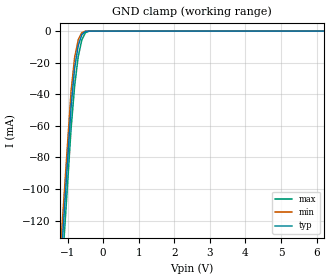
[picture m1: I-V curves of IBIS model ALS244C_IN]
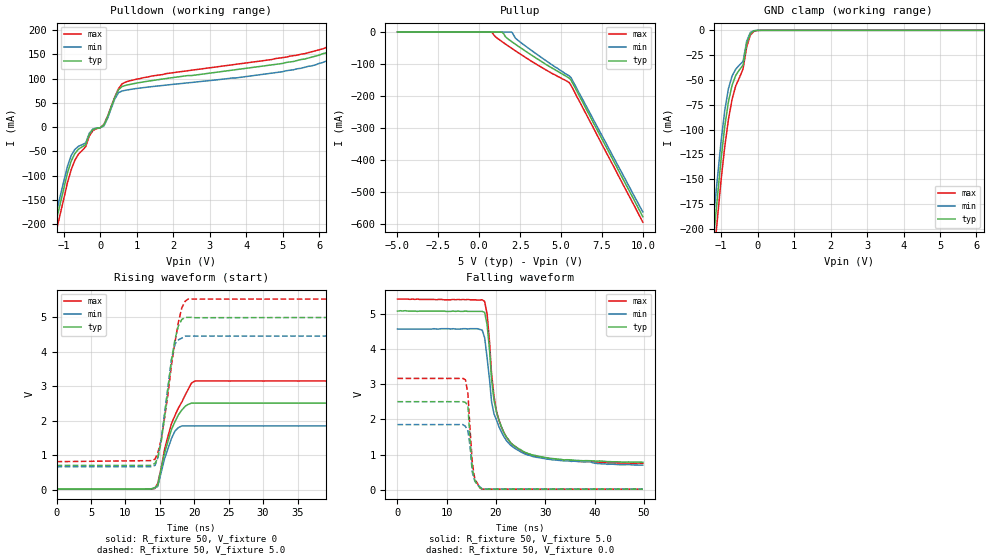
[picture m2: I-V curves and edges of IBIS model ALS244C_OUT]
| TEXAS INSTRUMENTS INCORPORATED
| Standard Linear and Logic Group
| IBIS Model of SN74ALS244C
| OCTAL BUFFERS AND LINE DRIVERS WITH 3-STATE OUTPUTS
| SOIC 20-pin (DW), SOP 20-pin (NS), SSOP 20-pin (DB), PDIP 20-pin (N) Package
[IBIS Ver]   3.2
[Comment Char]  |_char
[File Name]   sn74als244c.ibs
[File Rev]   3.1
[Date]   Sept. 23, 2004
[Source]   Data created from Labo data at TI-SLL.
[Notes]   The following is an IBIS list for the ALS244C.
   - FILE REV HISTORY
   - 3.1 Re-Release IBIS file on 09/23/04
   - Power clamp data deleted as there is no power-clamp diode
|   Please contact sllibis@ti.com with questions and
|   comments concerning SLL IBIS models.
[Disclaimer] Property of Texas Instruments Incorporated.  Unauthorized
   reproduction and/or distribution is strictly prohibited.
   This product is protected under copyright law.
   Created 2000, (C) Copyright 2000, Texas Instruments Inc.,
   All Rights Reserved.
   UNLESS THERE IS A SIGNED, WRITTEN AGREEMENT TO THE
   CONTRARY, TEXAS INSTRUMENTS () IS PROVIDING THE IBIS
   MODELS  AND WITHOUT ANY WARRANTY, EXPRESSED OR
   IMPLIED.  TI assumes no liability for:
   1) the accuracy of the IBIS models provided to your
   company;
   2) the proper functioning of these IBIS Models in your
   design or for any resulting applications; or
   3) infringement of patents, copyrights or intellectual
   property rights resulting from your use of these IBIS
   models.
   TI provides IBIS Models as a service to our customers.
   You and your company shall not distribute, sell or give
   these models to anyone else without prior written
   permission from TI.
   TI reserves the right to make changes to our products or
   to discontinue any semiconductor product or service
   without notice, and advises our customers to obtain the
   latest version of relevant information to verify, before
   placing orders, that the information being relied on is
   current.
   Please be aware that your receipt and use of the IBIS
   information provided shall serve as acceptance of these
   terms and conditions.  If you do not accept these terms,
   you should return or destroy the IBIS models and any
   other accompanying information immediately.
|   Component ALS244C_DW
[Component]   ALS244C_DW
[Manufacturer]  Texas Instruments, Inc.
[Package]
|   typ   min   max
R_pkg   0.038   0.033   0.045
L_pkg   5.012nH   4.110nH   6.349nH
C_pkg   0.717pF   0.530pF   0.868pF
[Pin]   signal_name   model_name   R_pin   L_pin   C_pin
1   1OE_NOT   ALS244C_IN   0.042   6.336nH   0.865pF
2   1A1   ALS244C_IN   0.043   5.542nH   0.867pF
3   2Y4   ALS244C_OUT   0.034   4.714nH   0.732pF
4   1A2   ALS244C_IN   0.034   4.377nH   0.591pF
5   2Y3   ALS244C_OUT   0.036   4.130nH   0.533pF
6   1A3   ALS244C_IN   0.035   4.111nH   0.530pF
7   2Y2   ALS244C_OUT   0.034   4.284nH   0.583pF
8   1A4   ALS244C_IN   0.034   4.634nH   0.726pF
9   2Y1   ALS244C_OUT   0.040   5.518nH   0.865pF
10   GND   GND   0.043   6.349nH   0.866pF
11   2A1   ALS244C_IN   0.041   6.281nH   0.861pF
12   1Y4   ALS244C_OUT   0.045   5.561nH   0.868pF
13   2A2   ALS244C_IN   0.033   4.778nH   0.742pF
14   1Y3   ALS244C_OUT   0.035   4.414nH   0.596pF
15   2A3   ALS244C_IN   0.035   4.110nH   0.533pF
16   1Y2   ALS244C_OUT   0.036   4.130nH   0.533pF
17   2A4   ALS244C_IN   0.034   4.377nH   0.591pF
18   1Y1   ALS244C_OUT   0.034   4.714nH   0.731pF
19   2OE_NOT   ALS244C_IN   0.043   5.569nH   0.868pF
20   VCC   POWER   0.042   6.308nH   0.864pF
|   Component ALS244C_NS
[Component]   ALS244C_NS
[Manufacturer]  Texas Instruments, Inc.
[Package]
|   typ   min   max
R_pkg   0.044   0.029   0.058
L_pkg   3.666nH   2.317nH   5.115nH
C_pkg   0.548pF   0.316pF   0.725pF
[Pin]   signal_name   model_name   R_pin   L_pin   C_pin
1   1OE_NOT   ALS244C_IN   0.058   5.115nH   0.725pF
2   1A1   ALS244C_IN   0.053   4.591nH   0.724pF
3   2Y4   ALS244C_OUT   0.049   3.754nH   0.572pF
4   1A2   ALS244C_IN   0.029   2.549nH   0.388pF
5   2Y3   ALS244C_OUT   0.031   2.317nH   0.316pF
6   1A3   ALS244C_IN   0.031   2.317nH   0.316pF
7   2Y2   ALS244C_OUT   0.029   2.556nH   0.399pF
8   1A4   ALS244C_IN   0.049   3.754nH   0.579pF
9   2Y1   ALS244C_OUT   0.053   4.591nH   0.724pF
10   GND   GND   0.058   5.115nH   0.725pF
11   2A1   ALS244C_IN   0.058   5.115nH   0.725pF
12   1Y4   ALS244C_OUT   0.053   4.591nH   0.724pF
13   2A2   ALS244C_IN   0.049   3.754nH   0.579pF
14   1Y3   ALS244C_OUT   0.029   2.557nH   0.399pF
15   2A3   ALS244C_IN   0.031   2.317nH   0.316pF
16   1Y2   ALS244C_OUT   0.031   2.317nH   0.316pF
17   2A4   ALS244C_IN   0.029   2.557nH   0.399pF
18   1Y1   ALS244C_OUT   0.049   3.754nH   0.579pF
19   2OE_NOT   ALS244C_IN   0.053   4.591nH   0.724pF
20   VCC   POWER   0.058   5.115nH   0.725pF
|   Component ALS244C_DB
[Component]   ALS244C_DB
[Manufacturer]  Texas Instruments, Inc.
[Package]
|   typ   min   max
R_pkg   0.040   0.035   0.051
L_pkg   3.495nH   3.035nH   4.314nH
C_pkg   0.420pF   0.346pF   0.502pF
[Pin]   signal_name   model_name   R_pin   L_pin   C_pin
1   1OE_NOT   ALS244C_IN   0.049   4.310nH   0.502pF
2   1A1   ALS244C_IN   0.048   3.903nH   0.487pF
3   2Y4   ALS244C_OUT   0.035   3.189nH   0.396pF
4   1A2   ALS244C_IN   0.035   3.036nH   0.347pF
5   2Y3   ALS244C_OUT   0.035   3.035nH   0.367pF
6   1A3   ALS244C_IN   0.035   3.035nH   0.367pF
7   2Y2   ALS244C_OUT   0.035   3.036nH   0.347pF
8   1A4   ALS244C_IN   0.035   3.189nH   0.397pF
9   2Y1   ALS244C_OUT   0.047   3.899nH   0.488pF
10   GND   GND   0.051   4.314nH   0.500pF
11   2A1   ALS244C_IN   0.051   4.314nH   0.500pF
12   1Y4   ALS244C_OUT   0.047   3.899nH   0.488pF
13   2A2   ALS244C_IN   0.035   3.189nH   0.397pF
14   1Y3   ALS244C_OUT   0.035   3.036nH   0.346pF
15   2A3   ALS244C_IN   0.035   3.035nH   0.367pF
16   1Y2   ALS244C_OUT   0.035   3.035nH   0.367pF
17   2A4   ALS244C_IN   0.035   3.036nH   0.346pF
18   1Y1   ALS244C_OUT   0.035   3.189nH   0.397pF
19   2OE_NOT   ALS244C_IN   0.047   3.899nH   0.488pF
20   VCC   POWER   0.051   4.314nH   0.502pF
|   Component ALS244C_N
[Component]   ALS244C_N
[Manufacturer]   Texas Instruments, Inc.
[Package]
|   typ   min   max
R_pkg   4.300e-02   3.800e-02   5.000e-02
L_pkg   7.384e-09   4.680e-09   1.032e-08
C_pkg   5.100e-13   2.310e-13   8.210e-13
[Pin]   signal_name   model_name   R_pin   L_pin   C_pin
1   1OE_NOT   ALS244C_IN   4.200e-02   9.427e-09   8.100e-13
2   1A1   ALS244C_IN   4.600e-02   8.544e-09   4.560e-13
3   2Y4   ALS244C_OUT   4.800e-02   7.163e-09   4.350e-13
4   1A2   ALS244C_IN   4.000e-02   4.825e-09   2.610e-13
5   2Y3   ALS244C_OUT   4.000e-02   5.284e-09   6.480e-13
6   1A3   ALS244C_IN   4.000e-02   4.686e-09   2.320e-13
7   2Y2   ALS244C_OUT   4.000e-02   6.359e-09   4.890e-13
8   1A4   ALS244C_IN   3.800e-02   7.982e-09   4.750e-13
9   2Y1   ALS244C_OUT   4.300e-02   9.403e-09   4.750e-13
10   GND   GND   5.000e-02   1.032e-08   8.050e-13
11   2A1   ALS244C_IN   5.000e-02   1.028e-08   8.100e-13
12   1Y4   ALS244C_OUT   4.300e-02   9.383e-09   4.770e-13
13   2A2   ALS244C_IN   3.800e-02   7.978e-09   4.760e-13
14   1Y3   ALS244C_OUT   4.000e-02   6.302e-09   4.920e-13
15   2A3   ALS244C_IN   4.000e-02   4.680e-09   2.310e-13
16   1Y2   ALS244C_OUT   4.000e-02   5.284e-09   6.480e-13
17   2A4   ALS244C_IN   4.000e-02   4.822e-09   2.610e-13
18   1Y1   ALS244C_OUT   4.700e-02   7.118e-09   4.390e-13
19   2OE_NOT   ALS244C_IN   4.600e-02   8.492e-09   4.610e-13
20   VCC   POWER   4.300e-02   9.348e-09   8.210e-13
| Models and submodels in the file (2): ALS244C_IN (Input), ALS244C_OUT (3-state)
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|   Model ALS244C_IN
[Model]   ALS244C_IN
Model_type  Input
Polarity   Non-Inverting
Vinl = 0.8
Vinh = 2.0
| variable   typ   min   max
C_comp   1.33pf   1.00pf   1.66pf
[Temperature Range]   25   0   70
[Voltage Range]   5.0   4.5   5.5
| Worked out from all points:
|   GND clamp passes 1 mA (typ) near -0.54 V on its own axis
[GND Clamp]
|   Voltage   I(typ)   I(min)   I(max)
-5V       -1.46A     -1.41A     -1.52A
-1.2V     -151mA     -138mA     -168mA
-1.1V     -117mA     -105mA     -132mA
-1V       -82.2mA    -71.2mA    -96.9mA
-900mV    -47.7mA    -37.7mA    -61.4mA
-800mV    -23.3mA    -16.5mA    -34.4mA
-700mV    -9.09mA    -5.49mA    -16.1mA
-600mV    -2.32mA    -965uA     -5.65mA
-500mV    -207uA     -49.9uA    -1.1mA
-400mV    -20.2uA    -16uA      -84.4uA
-300mV    -13.8uA    -14.7uA    -15.1uA
10V       2.13nA     225pA      4.62nA
|   Model ALS244C_OUT
[Model]   ALS244C_OUT
Model_type  3-state
Polarity   Non-Inverting
Enable   Active-Low
Vmeas = 2.5v
Cref = 15pf
| variable   typ   min   max
C_comp   5.8pf   4.35pf   7.25pf
[Temperature Range]   25   0   70
[Voltage Range]   5.0   4.5   5.5
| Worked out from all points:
|   slope of the pulldown table from 0 to 0.75 V, typ, clamps not added: 8.52 ohm
|   GND clamp passes 1 mA (typ) near -0.11 V on its own axis
|   rising waveform, R_fixture 50, V_fixture 0: 20-80 % time 2.21ns typ, 1.63ns min, 2.94ns max; typ from 0.021 V to 2.51 V
|   falling waveform, R_fixture 50, V_fixture 5.0: 20-80 % time 3.03ns typ, 3.61ns min, 2.9ns max; typ from 5.07 V to 0.782 V
|   rising waveform, R_fixture 50, V_fixture 5.0: 20-80 % time 1.7ns typ, 1.46ns min, 2.03ns max; typ from 0.706 V to 4.99 V
|   falling waveform, R_fixture 50, V_fixture 0.0: 20-80 % time 832ps typ, 914ps min, 943ps max; typ from 2.5 V to 0.019 V
[Pulldown]
|   Voltage   I(typ)   I(min)   I(max)
-5V       -1.4A      -1.34A     -1.44A
-1.4V     -254mA     -234mA     -276mA
-1.2V     -190mA     -173mA     -212mA
-900mV    -94.5mA    -80.4mA    -114mA
-700mV    -54.5mA    -46.1mA    -68.4mA
-200mV    -4.82mA    -3.55mA    -6.79mA
100mV     4.21mA     2.48mA     5.91mA
500mV     76.9mA     70.9mA     79.1mA
700mV     86mA       75.9mA     92.9mA
5.8V      144mA      126mA      155mA
7.6V      239mA      228mA      252mA
10V       425mA      436mA      450mA
[Pullup]
|   Voltage   I(typ)   I(min)   I(max)
-5V       18.8nA     1.71nA     273nA
700mV     18.8nA     1.71nA     -78.4uA
800mV     18.8nA     1.71nA     -1.62mA
1V        18.8nA     1.71nA     -15mA
1.4V      -389uA     1.71nA     -30.2mA
1.6V      -14.4mA    1.69nA     -37.3mA
2V        -30.5mA    -634uA     -51.3mA
2.2V      -37.6mA    -18.3mA    -58.2mA
2.6V      -51.7mA    -35mA      -71.7mA
5.5V      -144mA     -137mA     -158mA
5.7V      -159mA     -151mA     -175mA
10V       -578mA     -563mA     -595mA
[GND Clamp]
|   Voltage   I(typ)   I(min)   I(max)
-5V       -1.67A     -1.58A     -1.72A
-1.3V     -245mA     -222mA     -268mA
-1.2V     -206mA     -185mA     -228mA
-1.1V     -167mA     -148mA     -189mA
-900mV    -96.5mA    -80.3mA    -117mA
-800mV    -71.9mA    -58.7mA    -89.6mA
-600mV    -45.4mA    -39.1mA    -55.9mA
-400mV    -35mA      -31.3mA    -38.8mA
-300mV    -13.4mA    -11.1mA    -16.7mA
-200mV    -3.29mA    -2.13mA    -4.83mA
-100mV    -596uA     -308uA     -1.06mA
10V       3.02nA     210pA      25.3nA
[Ramp]
| variable   typ   min   max
dV/dt_r   1.52E+00/2.32E-09   1.31E+00/2.29E-09   1.70E+00/2.40E-09
dV/dt_f   2.63E+00/3.12E-09   2.33E+00/3.42E-09   2.86E+00/2.98E-09
R_load = 50
[Rising Waveform]
R_fixture = 50
V_fixture = 0
|   Time   V(typ)   V(min)   V(max)
0s        20.9mV     20.5mV     20.2mV
14.3ns    69.6mV     56.8mV     40.8mV
14.7ns    133mV      98.1mV     191mV
15.7ns    1.07V      908mV      1.18V
16.7ns    1.75V      1.49V      1.92V
17.2ns    1.97V      1.7V       2.15V
18.7ns    2.42V      1.85V      2.75V
19.6ns    2.51V      1.85V      3.09V
20.1ns    2.51V      1.85V      3.15V
49.8ns    2.51V      1.85V      3.15V
[Falling Waveform]
R_fixture = 50
V_fixture = 5.0
V_fixture_min = 4.5
V_fixture_max = 5.5
|   Time   V(typ)   V(min)   V(max)
0s        5.07V      4.56V      5.41V
16.2ns    5.06V      4.57V      5.38V
17.7ns    5.03V      4.31V      5.34V
18.2ns    4.68V      3.74V      4.98V
19.1ns    3.13V      2.5V       3.29V
20.1ns    2.2V       1.98V      2.23V
22.1ns    1.5V       1.4V       1.5V
25ns      1.14V      1.08V      1.12V
33.8ns    849mV      821mV      837mV
49.8ns    782mV      702mV      754mV
[Rising Waveform]
R_fixture = 50
V_fixture = 5.0
V_fixture_min = 4.5
V_fixture_max = 5.5
|   Time   V(typ)   V(min)   V(max)
0s        706mV      670mV      816mV
14.3ns    769mV      707mV      890mV
14.7ns    918mV      916mV      1.06V
15.2ns    1.39V      1.45V      1.45V
16.2ns    2.93V      3.01V      2.79V
16.7ns    3.75V      3.79V      3.62V
17.2ns    4.35V      4.22V      4.26V
18.2ns    4.93V      4.39V      5.27V
19.1ns    4.99V      4.45V      5.52V
49.8ns    4.99V      4.45V      5.52V
[Falling Waveform]
R_fixture = 50
V_fixture = 0.0
|   Time   V(typ)   V(min)   V(max)
0s        2.5V       1.85V      3.16V
13.3ns    2.5V       1.85V      3.16V
13.8ns    2.48V      1.8V       3.12V
14.3ns    2.39V      1.67V      2.73V
14.7ns    1.48V      1.27V      1.79V
15.2ns    577mV      488mV      767mV
15.7ns    273mV      246mV      299mV
16.7ns    67.1mV     89.5mV     58.3mV
17.2ns    19.2mV     27.6mV     19.2mV
49.8ns    19.2mV     27.6mV     19.2mV
